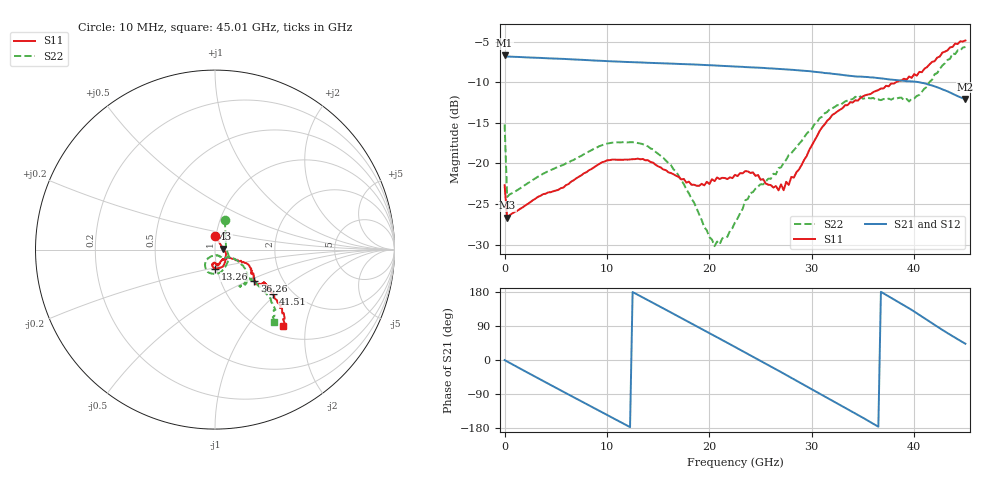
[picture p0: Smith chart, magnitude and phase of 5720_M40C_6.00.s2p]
! Device:  ADRF5720
! Description: 0.5dB LSB GaAs MMIC 6-bit Digital Attenuator
! Frequency:  0.000009 -  40 GHz
! Ports:
!	RF1	= Port 1
!	RF2	= Port 2
! Vdd:  3.3 Volt
! Vss:  -3.3 Volt
! Control:  0/3.3 Volt
! State:  6.00 dB attenuation
! Data:  The device was measured using G-S-G Probes on a matrix board.
!  Data was collected using an calibrated 4 port network analyzer.
!  The reference plane for this measurement is at the launchers.
! Note:  Analog Devices supplies this data as a sample of measured data
!  for this product.  Your particular data for this product may vary.
!  Data was taken at -40 degrees C.
!  Analog Devices reserves the right to change this data at anytime.
# GHZ S DB R 45.0
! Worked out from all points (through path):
!   181 points, 10 MHz to 45.01 GHz, reference 45 ohm
!   highest |S21| = -6.68 dB at 10 MHz (marker M1); lowest = -12.1 dB at 45.01 GHz (marker M2)
!   group delay of S21, straight-line fit = 41.3 ps
!   lowest |S11| = -26.7 dB at 260 MHz (marker M3), VSWR 1.10, Z = 49.3 + j0.589 ohm
!   |S11| at or under -10 dB: start of sweep to 38.25 GHz
!   |S22| runs from -30.2 to -5.7 dB; largest |S21 - S12| = 0.0018
!   S11 on the Smith chart (normalised r, x): 10 MHz: 0.99, +0.15; 13.26 GHz: 0.98, -0.21; 36.26 GHz: 1.44, -0.54; 41.51 GHz: 1.60, -0.95; 45.01 GHz: 1.20, -1.51
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0.01  -22.70 88.6  -6.68 -0.3  -6.70 -0.3  -15.22 71.7
0.26  -26.70 7.4  -6.85 -4.0  -6.86 -4.0  -24.14 4.3
2.01  -25.21 -9.3  -6.94 -29.7  -6.96 -29.8  -22.67 -14.5
4.26  -23.58 -21.2  -7.07 -62.4  -7.09 -62.4  -20.96 -31.5
6.01  -22.68 -35.5  -7.16 -87.6  -7.18 -87.6  -20.00 -46.1
7.76  -21.22 -48.8  -7.27 -112.8  -7.28 -112.8  -18.87 -61.3
10.76  -19.55 -70.0  -7.45 -155.7  -7.47 -155.7  -17.46 -85.5
13.26  -19.51 -89.7  -7.58 168.6  -7.60 168.6  -17.56 -105.4
15.26  -20.51 -98.2  -7.67 139.8  -7.68 139.8  -19.06 -119.5
18.01  -22.25 -96.9  -7.81 100.1  -7.83 100.0  -23.71 -129.7
20.51  -22.19 -86.6  -7.95 63.7  -7.97 63.6  -30.20 -87.3
22.76  -21.57 -83.9  -8.09 30.8  -8.12 30.7  -26.79 -53.5
23.51  -20.96 -79.1  -8.15 19.9  -8.17 19.7  -24.55 -50.1
25.01  -22.02 -72.0  -8.23 -2.2  -8.25 -2.4  -22.57 -37.8
27.26  -23.31 -49.9  -8.41 -35.7  -8.43 -35.9  -19.95 -25.7
30.26  -17.23 -24.4  -8.72 -81.0  -8.74 -81.2  -15.21 -29.9
32.76  -13.41 -25.8  -9.07 -118.8  -9.10 -118.9  -12.85 -39.5
36.26  -11.09 -38.4  -9.47 -172.2  -9.50 -172.3  -12.16 -54.4
37.76  -10.17 -39.1  -9.69 164.2  -9.72 164.1  -12.16 -54.9
39.51  -9.31 -34.4  -9.90 136.4  -9.92 136.2  -12.38 -42.9
41.51  -7.80 -37.5  -10.34 101.4  -10.36 101.2  -9.97 -39.8
45.01  -4.87 -48.1  -12.09 42.9  -12.12 42.8  -5.68 -50.6
